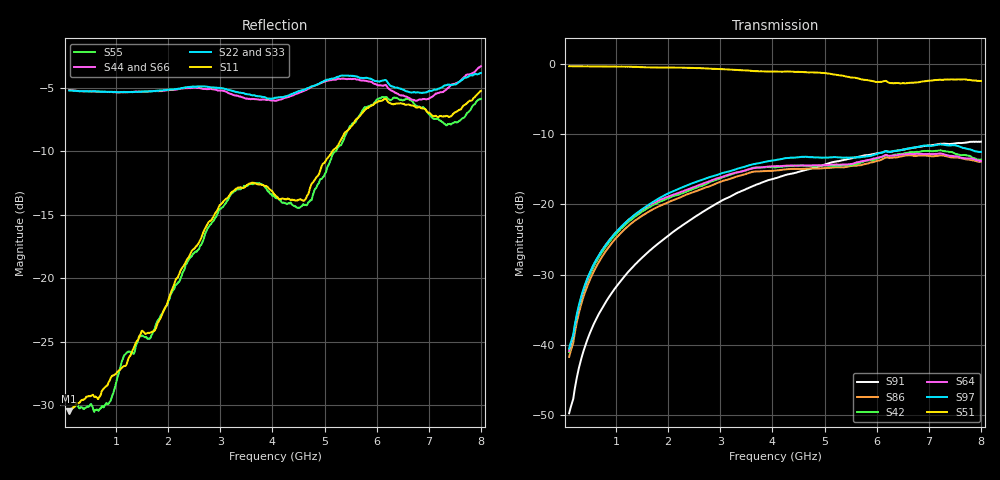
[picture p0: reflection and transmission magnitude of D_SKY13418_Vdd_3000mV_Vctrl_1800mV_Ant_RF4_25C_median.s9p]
# GHz S DB R 50
! THRU S21 mag phase subtraction.
! HALF_THRU
! EN33-165-011-v1_HALF_THRU_1 EN33-165-011-v1_HALF_THRU_2 EN33-165-011-v1_HALF_THRU_3 EN33-165-011-v1_HALF_THRU_4 EN33-165-011-v1_HALF_THRU_5 EN33-165-011-v1_HALF_THRU_6 EN33-165-011-v1_HALF_THRU_7 EN33-165-011-v1_HALF_THRU_8 EN33-165-011-v1_HALF_THRU_9
! THRU Ports: 1 2
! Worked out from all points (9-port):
!   801 points, 100 MHz to 8 GHz, reference 50 ohm
!   strongest paths, dB at 100 MHz, 2.075 GHz, 4.05 GHz, 6.025 GHz, 8 GHz:
!     S51: -0.4, -0.6, -1.1, -2.6, -2.5
!     S97: -40.5, -18.2, -13.7, -12.8, -12.5
!     S64: -40.8, -18.7, -14.6, -13.4, -13.8
!     S42: -41.0, -18.9, -14.7, -13.5, -13.6
!     S86: -41.7, -19.5, -15.2, -13.8, -14.0
!     S91: -49.7, -24.0, -16.3, -12.7, -11.1
!   lowest |S11| = -30.5 dB at 100 MHz (marker M1), VSWR 1.06, Z = 53.1 + j0.146 ohm
!   |S11| at or under -10 dB: start of sweep to 5.151 GHz
